// 轴对象
FUNCTION_BLOCK FB_NcAxis EXTENDS Tc2_MC2.AXIS_REF 
VAR
	{attribute ‘hide’}
	mcReadStatus	         :Tc2_MC2.MC_ReadStatus;	
	{attribute ‘hide’}
	mcReadActPos	         :Tc2_MC2.MC_ReadActualPosition;
	{attribute ‘hide’}
	mcReadActVel             :Tc2_MC2.MC_ReadActualVelocity;
	{attribute ‘hide’}
	mcPower                  :Tc2_MC2.MC_Power;
	{attribute ‘hide’}
	mcMoveRel		         :Tc2_MC2.MC_MoveRelative;
	{attribute ‘hide’}
	mcMoveAbs		         :Tc2_MC2.MC_MoveAbsolute;
	{attribute ‘hide’}
	mcMoveVelocity           :Tc2_MC2.MC_MoveVelocity;
	{attribute ‘hide’}
	mcMoveModulo			 :Tc2_MC2.MC_MoveModulo;
	{attribute ‘hide’}
	mcReset                  :Tc2_MC2.MC_Reset;
	{attribute ‘hide’}
	mcJogContinous           :Tc2_MC2.MC_Jog;
	{attribute ‘hide’}
	mcJogRelative            :Tc2_MC2.MC_Jog;
	{attribute ‘hide’}
	mcStop                   :Tc2_MC2.MC_Stop;
	{attribute ‘hide’}
	mcHalt                   :Tc2_MC2.MC_Halt;
	{attribute ‘hide’}
	mcsetOverride            :Tc2_MC2.MC_SetOverride;

	mchome					 :Tc2_Mc2.MC_Home;
	
	_NCTOPLC				 : NCTOPLC_AXIS_REF;

	
END_VAR

PROPERTY AxesStatus : REFERENCE TO Tc2_Mc2.ST_AxisStatus
GET
AxesStatus	REF= Status;
END_GET
END_PROPERTY

// 刷新状态
METHOD PUBLIC CyclicCheck
VAR_INPUT
END_VAR
ReadStatus();
_NCTOPLC	:= NCTOPLC;
END_METHOD

// 暂停
METHOD Halt : BOOL
VAR_INPUT
	Execute              :BOOL;
END_VAR
mcHalt(
	Axis:=THIS^ , 
	Execute:=Execute , 
	Deceleration:=800000 , 
	Jerk:=80000 , 
	BufferMode:= , 
	Options:= , 
	Done=> , 
	Busy=> , 
	Active=> , 
	CommandAborted=> , 
	Error=>Status.Error , 
	ErrorID=>Status.ErrorId );
	
IF mcHalt.Done AND NOT Status.Error THEN
	Halt := TRUE;
ELSE
	Halt := FALSE;
END_IF
END_METHOD

// 绝对定位
METHOD MoveAbs : BOOL
VAR_INPUT
	Execute             :BOOL;
	TargetPos:REAL;
	TargetVel         :ST_axis_Vel;
END_VAR
mcMoveAbs(
	Axis:= THIS^, 
	Execute:= Execute, 
	Position:= TargetPos, 
	Velocity:= TargetVel.Axis_Vel, 
	Acceleration:= TargetVel.Axis_Acc, 
	Deceleration:= TargetVel.Axis_Dec, 
	Jerk:= TargetVel.Axis_Jerk, 
	BufferMode:= , 
	Options:= , 
	Done=> , 
	Busy=> , 
	Active=> , 
	CommandAborted=> , 
	Error=>Status.Error , 
	ErrorID=>Status.ErrorId );
	
IF mcMoveAbs.Done AND NOT Status.Error THEN
	MoveAbs := TRUE;
ELSE
	MoveAbs := FALSE;
END_IF
END_METHOD

// 点动
METHOD MoveJog : BOOL
VAR_INPUT
	JogForward                 :BOOL;
	JogBackwards               :BOOL;
	TargetVel       :LREAL;
END_VAR
mcJogContinous(
	JogForward:= 	JogForward,
	JogBackwards:= 	JogBackwards,
	Mode:= 			MC_JOGMODE_CONTINOUS,
	Velocity:= 		TargetVel,
	Axis:= 			THIS^,
	Error=>Status.Error , 
	ErrorID=>Status.ErrorId );
	
MoveJog:=mcJogContinous.Busy;
END_METHOD

// 速度运动
METHOD MoveVelocity : BOOL
VAR_INPUT
	Execute:BOOL;
	TargetVel       : ST_axis_Vel;
	Direction		: MC_Direction;
END_VAR
mcMoveVelocity(
	Axis:=THIS^ , 
	Execute:= Execute, 
	Velocity:= TargetVel.Axis_Vel, 
	Acceleration:= TargetVel.Axis_Acc, 
	Deceleration:= TargetVel.Axis_Dec, 
	Jerk:= TargetVel.Axis_Jerk, 
	Direction:= Direction, 
	BufferMode:= , 
	Options:= , 
	InVelocity=> , 
	Busy=> , 
	Active=> , 
	CommandAborted=> , 
	Error=>Status.Error , 
	ErrorID=> Status.ErrorId);
END_METHOD

PROPERTY NC_TO_PLC : REFERENCE TO Tc2_Mc2.NCTOPLC_AXIS_REF
GET
NC_TO_PLC	REF= _NcToPlc;
END_GET
END_PROPERTY

// 使能
METHOD Power : BOOL
VAR_INPUT
	Enable         :BOOL;
END_VAR
mcPower(
	Axis:= THIS^, 
	Enable:= Enable, 
	Enable_Positive:=TRUE, //NOT AxisSingle.Positive, 
	Enable_Negative:=TRUE, //NOT AxisSingle.Negtive, 
	Error=>Status.Error , 
	ErrorID=>Status.ErrorId );
END_METHOD

PROPERTY rAxis : REFERENCE TO Tc2_Mc2.AXIS_REF
GET
rAxis	REF= THIS^;
END_GET
END_PROPERTY

// 复位
METHOD Reset : BOOL
VAR_INPUT
	Execute              :BOOL;
END_VAR
mcReset(
	Axis:= THIS^, 
	Execute:=Execute , 
	Error=>Status.Error , 
	ErrorID=>Status.ErrorId );
	
IF NOT Status.Error	AND mcReset.Done THEN
	Reset	:= TRUE;
END_IF
END_METHOD

// 停止
METHOD Stop : BOOL
VAR_INPUT
	Execute              :BOOL;
END_VAR
mcStop(
	Axis:= THIS^, 
	Execute:=Execute , 
	Error=>Status.Error , 
	ErrorID=>Status.ErrorId );
	
	
IF NOT Status.Error	AND mcStop.Done THEN
	Stop	:= TRUE;
END_IF
END_METHOD

METHOD TestMode
VAR_INPUT
END_VAR
VAR
	
END_VAR
THIS^.CyclicCheck();

mcPower(
	Axis:= THIS^,
	Enable_Positive:=TRUE,
	Enable_Negative:=TRUE );
	
mcMoveAbs(Axis:= THIS^ );

mcReset(Axis:= THIS^);

mcStop(Axis:= THIS^);
END_METHOD

END_FUNCTION_BLOCK
